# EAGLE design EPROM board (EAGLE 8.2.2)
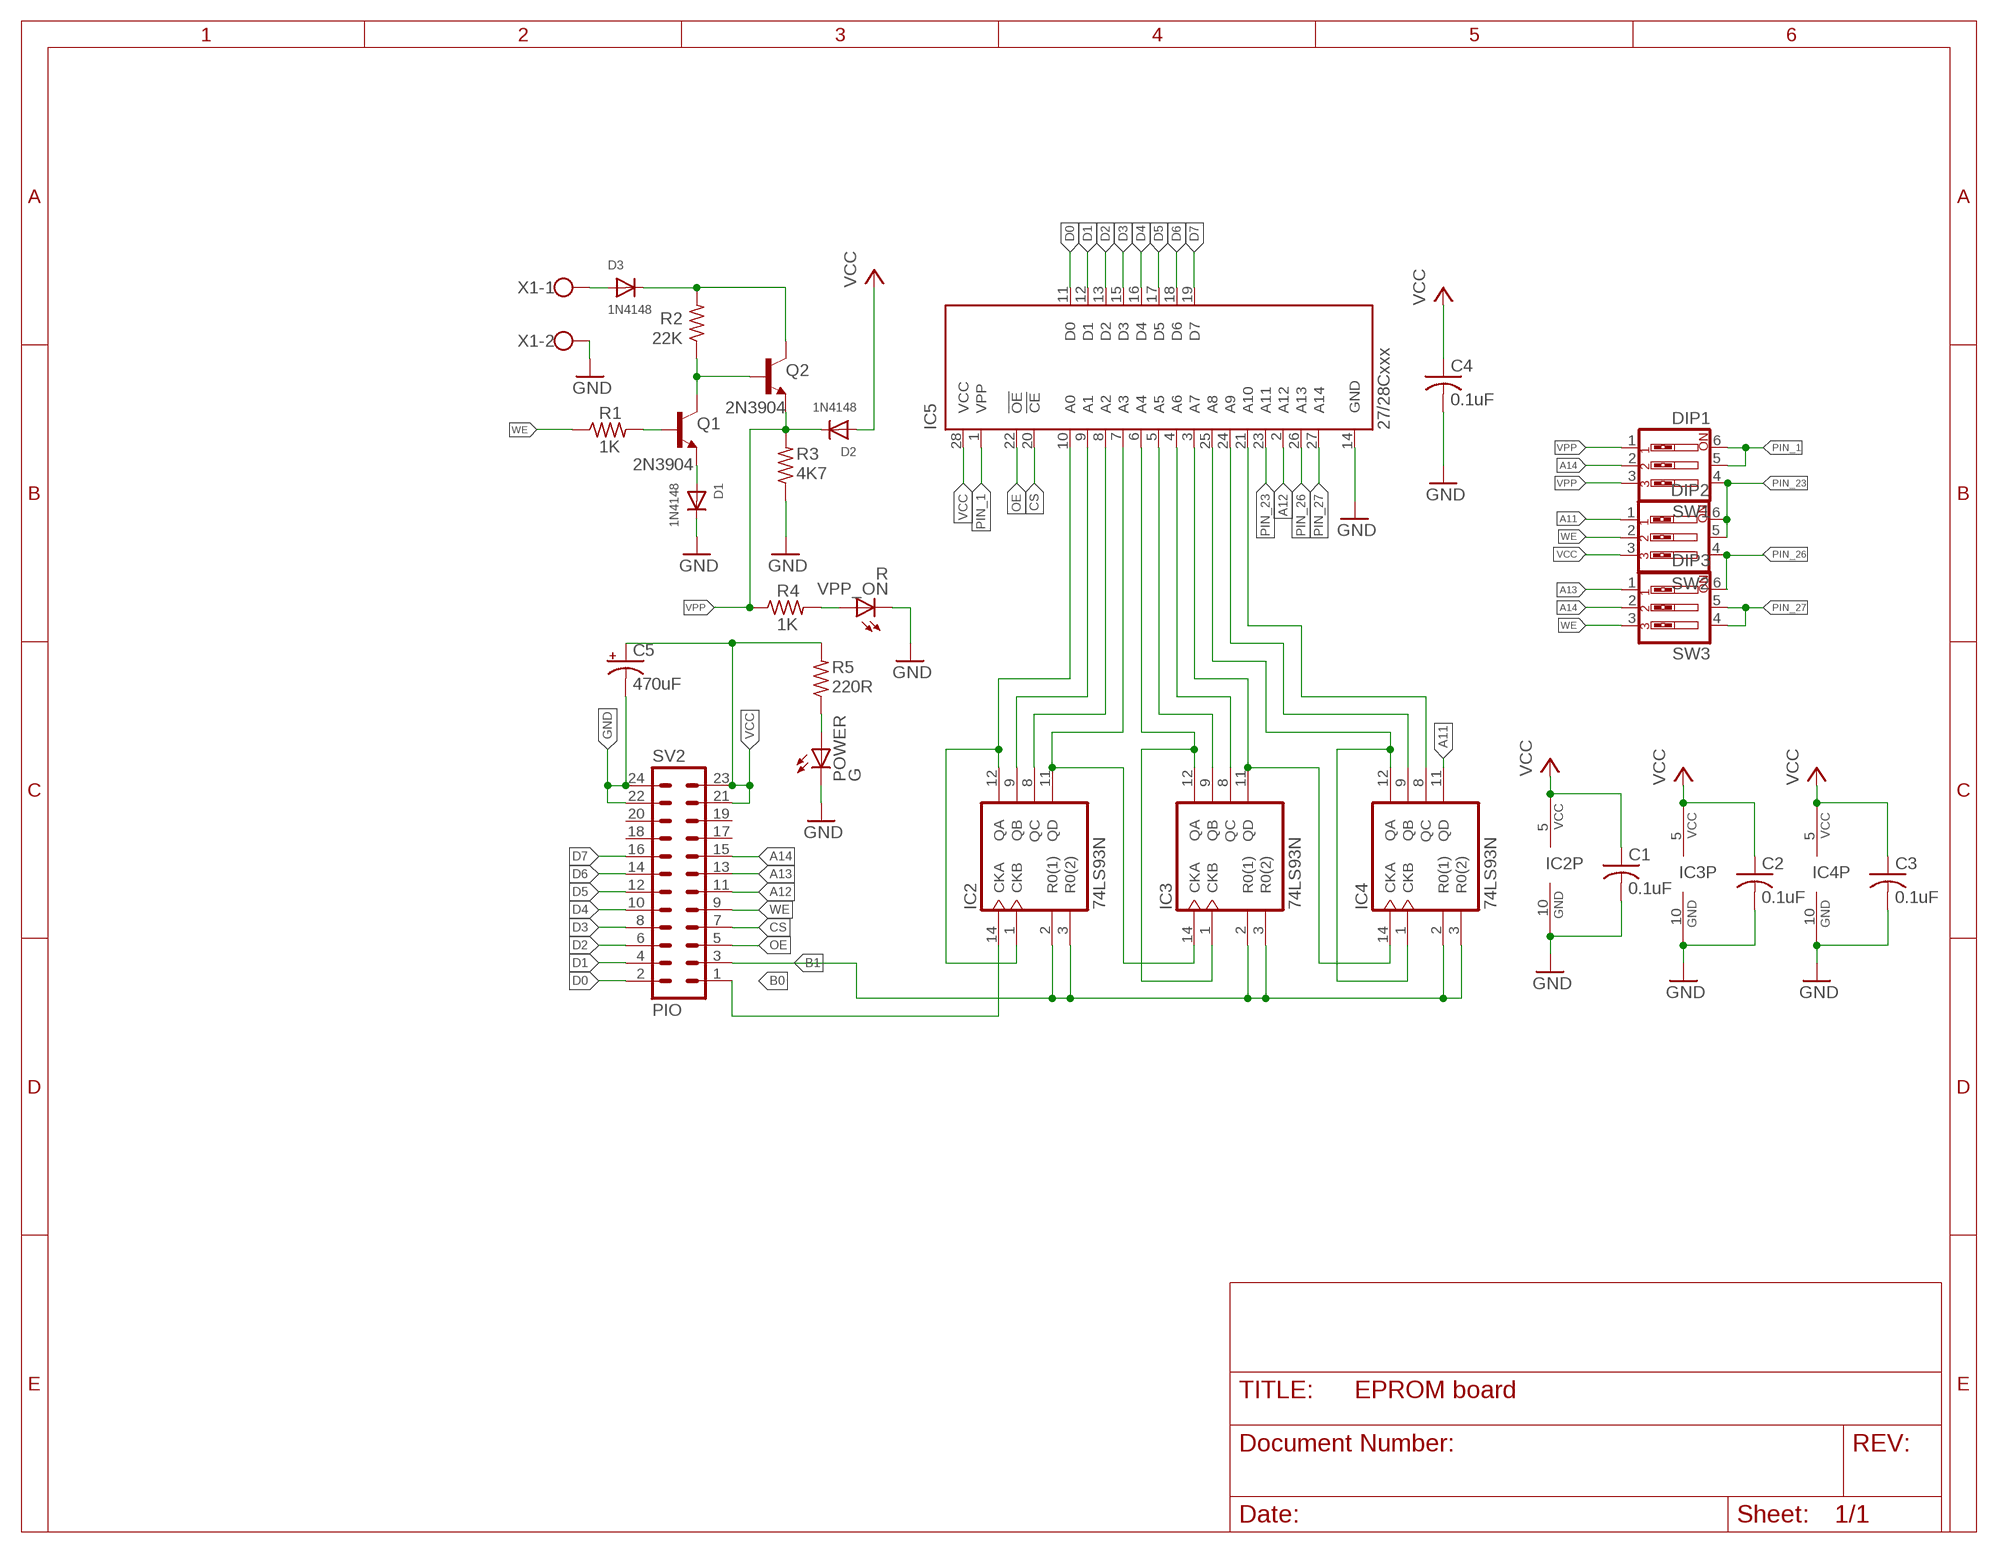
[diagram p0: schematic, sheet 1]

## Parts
C1  0.1uF  C-US025-025X050  [C025-025X050]
C2  0.1uF  C-US025-025X050  [C025-025X050]
C3  0.1uF  C-US025-025X050  [C025-025X050]
C4  0.1uF  C-US025-025X050  [C025-025X050]
C5  470uF  CPOL-USE5-6  [E5-6]
D1  1N4148  DIODEDO-1N4148  [DO-1N4148]
D2  1N4148  DIODEDO-1N4148  [DO-1N4148]
D3  1N4148  DIODEDO-1N4148  [DO-1N4148]
IC2  74LS93N  [DIL14]
IC3  74LS93N  [DIL14]
IC4  74LS93N  [DIL14]
IC5  27/28Cxxx  27C256P  [DIL28-6]
POWER  G  LED5MM  [LED5MM]
Q1  2N3904  [TO92]
Q2  2N3904  [TO92]
R1  1K  R-US_0204/7  [0204/7]
R2  22K  R-US_0204/7  [0204/7]
R3  4K7  R-US_0204/7  [0204/7]
R4  1K  R-US_0204/7  [0204/7]
R5  220R  R-US_0204/7  [0204/7]
SV2  PIO  MA12-2W  [MA12-2W]
SW1  DIP1  SW_DIP-3  [EDG-03]
SW2  DIP2  SW_DIP-3  [EDG-03]
SW3  DIP3  SW_DIP-3  [EDG-03]
VPP_ON  R  LED5MM  [LED5MM]
X1  W237-102  [W237-102]

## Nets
A11: IC4.11(QD) SW2.1
A12: IC5.2(A12) SV2.11
A13: SV2.13 SW3.1
A14: SV2.15 SW1.2 SW3.2
B0: IC2.14(CKA) SV2.1
B1: IC2.2(R0(1)) IC2.3(R0(2)) IC3.2(R0(1)) IC3.3(R0(2)) IC4.2(R0(1)) IC4.3(R0(2)) SV2.3
CS: IC5.20(!CE) SV2.7
D0: IC5.11(D0) SV2.2
D1: IC5.12(D1) SV2.4
D2: IC5.13(D2) SV2.6
D3: IC5.15(D3) SV2.8
D4: IC5.16(D4) SV2.10
D5: IC5.17(D5) SV2.12
D6: IC5.18(D6) SV2.14
D7: IC5.19(D7) SV2.16
GND: C1.2 C2.2 C3.2 C4.2 C5.- D1.C IC2.10(GND) IC3.10(GND) IC4.10(GND) IC5.14(GND) POWER.K(C) R3.1 SV2.22 SV2.24 VPP_ON.K(C) X1.2
N$1: IC2.1(CKB) IC2.12(QA) IC5.10(A0)
N$2: IC2.9(QB) IC5.9(A1)
N$3: IC2.8(QC) IC5.8(A2)
N$4: IC2.11(QD) IC3.14(CKA) IC5.7(A3)
N$5: IC3.1(CKB) IC3.12(QA) IC5.6(A4)
N$6: IC3.9(QB) IC5.5(A5)
N$7: IC3.8(QC) IC5.4(A6)
N$8: IC3.11(QD) IC4.14(CKA) IC5.3(A7)
N$9: IC4.1(CKB) IC4.12(QA) IC5.25(A8)
N$10: IC4.9(QB) IC5.24(A9)
N$11: IC4.8(QC) IC5.21(A10)
N$12: POWER.A R5.1
N$13: Q1.2(B) R1.2
N$14: D1.A Q1.3(E)
N$15: Q1.1(C) Q2.2(B) R2.1
N$16: D3.A X1.1
N$17: D3.C Q2.1(C) R2.2
N$18: R4.2 VPP_ON.A
OE: IC5.22(!OE) SV2.5
PIN_1: IC5.1(VPP) SW1.5 SW1.6
PIN_23: IC5.23(A11) SW1.4 SW2.5 SW2.6
PIN_26: IC5.26(A13) SW2.4 SW3.6
PIN_27: IC5.27(A14) SW3.4 SW3.5
VCC: C1.1 C2.1 C3.1 C4.1 C5.+ D2.A IC2.5(VCC) IC3.5(VCC) IC4.5(VCC) IC5.28(VCC) R5.2 SV2.21 SV2.23 SW2.3
VPP: D2.C Q2.3(E) R3.2 R4.1 SW1.1 SW1.3
WE: R1.1 SV2.9 SW2.2 SW3.3
Unconnected: SV2.17 SV2.18 SV2.19 SV2.20

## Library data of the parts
C1-C4 = rcl:C-US: CAPACITOR, American symbol
C5 = rcl:CPOL-US: POLARIZED CAPACITOR, American symbol
D1-D3 = adafruit:DIODE: Diode
IC2-IC4 = 74xx-us:74*93: Decade, divide by twelve and binary COUNTER
IC5 = microchip:27*256: CMOS EPROM 256 K (32 K x 8), low voltage; MF: Arrow Electronics; MPN: M27C256B15F1; OC_FARNELL: 1125431; OC_NEWARK: 93K7335
POWER VPP_ON = led:LED: LED
Q1 Q2 = transistor-npn:2N3904: NPN Transistor
R1-R5 = rcl:R-US_: RESISTOR, American symbol
SV2 = con-lstb:MA12-2W: PIN HEADER; OC_FARNELL: unknown; OC_NEWARK: unknown
SW1-SW3 = special:SW_DIP-3: DIP SWITCH
X1 = con-wago-500:W237-102: WAGO SCREW CLAMP; MPN: 237-102; OC_FARNELL: unknown; OC_NEWARK: 70K9898

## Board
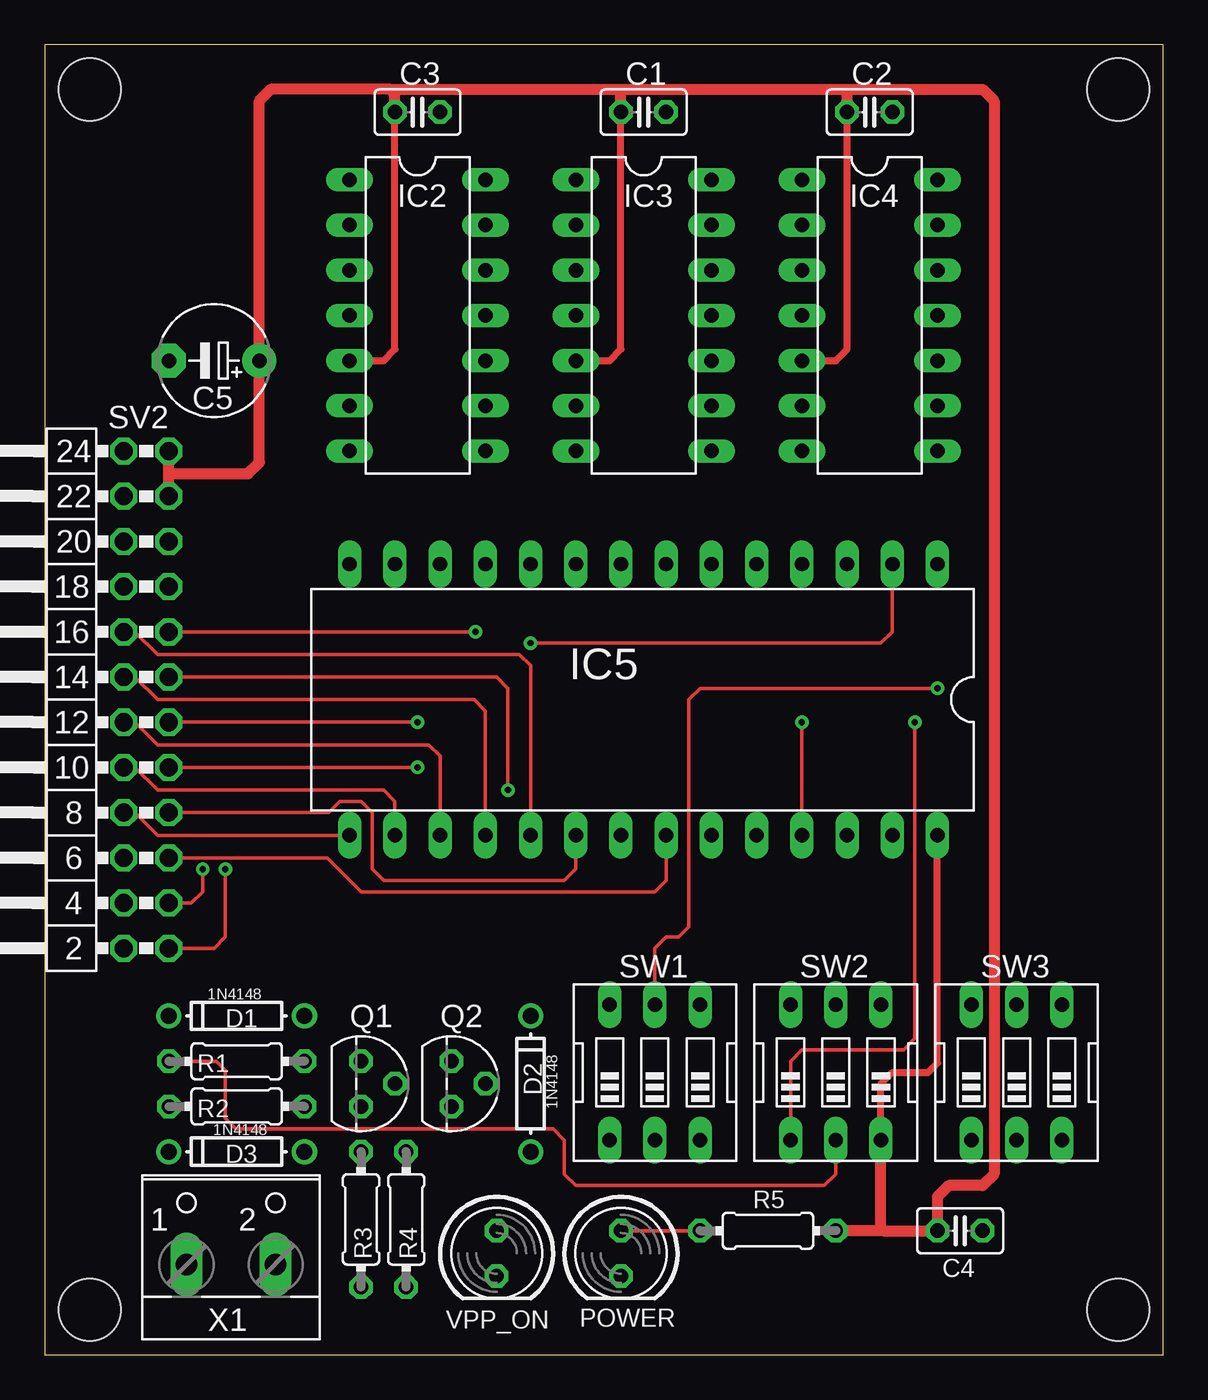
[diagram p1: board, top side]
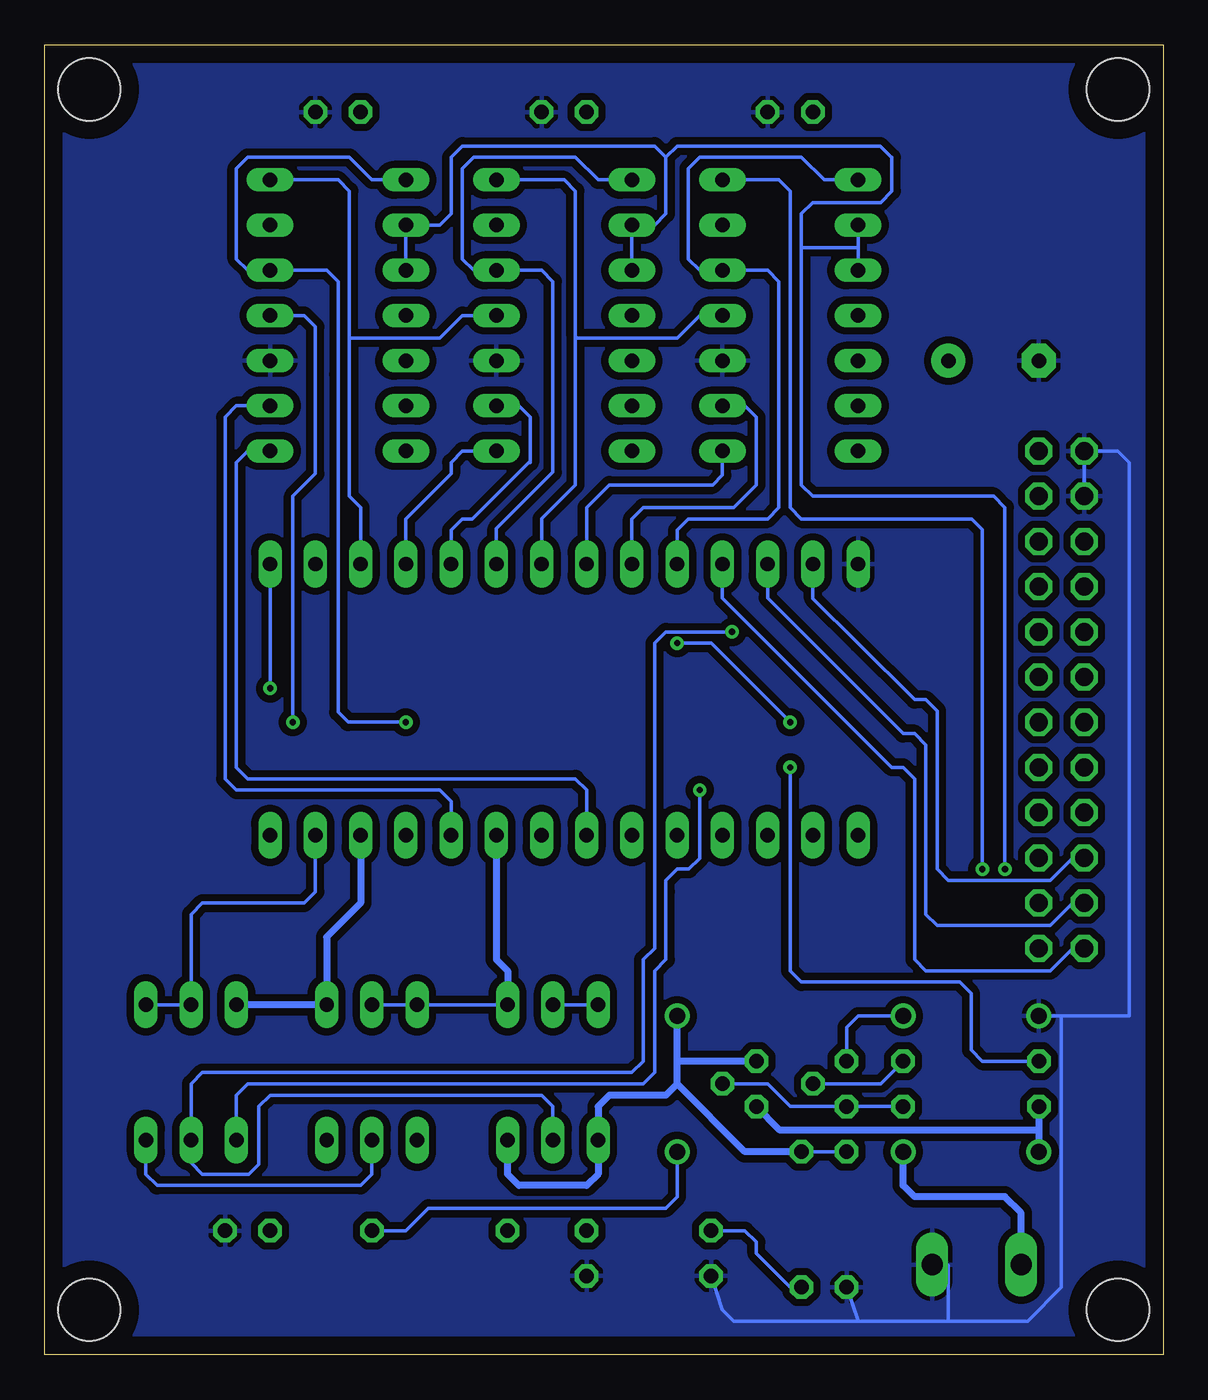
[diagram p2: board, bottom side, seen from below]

Size 62.84 x 73.65 mm. Coordinates in mm from the lower left corner, seen from the top.
Outline: 0,0 62.84,0 62.84,73.65 0,73.65 0,0
Copper layers (1*16): Top 0.035mm / dielectric 1.5mm / Bottom 0.035mm
Design rules "default": minimum track width 6mil, minimum drill 0.35mm, track to track 6mil, track to pad 6mil, pad to pad 6mil, via to via 6mil, smd to smd 6mil, copper to edge 40mil, drill to drill 6mil, minimum pad ring 10mil, minimum via ring 8mil, stop-mask expansion 4mil, vias tented up to drill 0mil, thermal gap 10mil
Holes 3.5 mm at 2.54,2.54 2.54,71.12 60.33,2.54 60.33,71.12

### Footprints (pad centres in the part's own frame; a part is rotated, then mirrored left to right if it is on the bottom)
C025-025X050 = drill 0.813 octagon: 1 -1.27,0; 2 1.27,0
E5-6 = drill 0.813 pad 1.905: + -2.54,0 | drill 0.813 pad 1.905 octagon: - 2.54,0
DO-1N4148 = drill 0.9: A -3.81,0; C 3.81,0
DIL14 = drill 0.813 long: 1 -7.62,-3.81; 2 -5.08,-3.81; 3 -2.54,-3.81; 4 0,-3.81; 5 2.54,-3.81; 6 5.08,-3.81; 7 7.62,-3.81; 8 7.62,3.81; 9 5.08,3.81; 10 2.54,3.81; 11 0,3.81; 12 -2.54,3.81; 13 -5.08,3.81; 14 -7.62,3.81
DIL28-6 = drill 0.813 long: 1 -16.51,-7.62; 2 -13.97,-7.62; 3 -11.43,-7.62; 4 -8.89,-7.62; 5 -6.35,-7.62; 6 -3.81,-7.62; 7 -1.27,-7.62; 8 1.27,-7.62; 9 3.81,-7.62; 10 6.35,-7.62; 11 8.89,-7.62; 12 11.43,-7.62; 13 13.97,-7.62; 14 16.51,-7.62; 15 16.51,7.62; 16 13.97,7.62; 17 11.43,7.62; 18 8.89,7.62; 19 6.35,7.62; 20 3.81,7.62; 21 1.27,7.62; 22 -1.27,7.62; 23 -3.81,7.62; 24 -6.35,7.62; 25 -8.89,7.62; 26 -11.43,7.62; 27 -13.97,7.62; 28 -16.51,7.62
LED5MM = drill 0.813 octagon: A -1.27,0; K 1.27,0
TO92 = drill 0.813 octagon: 1 1.27,0; 2 0,1.905; 3 -1.27,0
0204/7 = drill 0.813 octagon: 1 -3.81,0; 2 3.81,0
MA12-2W = drill 1.016 octagon: 1 -13.97,-1.27; 2 -13.97,1.27; 3 -11.43,-1.27; 4 -11.43,1.27; 5 -8.89,-1.27; 6 -8.89,1.27; 7 -6.35,-1.27; 8 -6.35,1.27; 9 -3.81,-1.27; 10 -3.81,1.27; 11 -1.27,-1.27; 12 -1.27,1.27; 13 1.27,-1.27; 14 1.27,1.27; 15 3.81,-1.27; 16 3.81,1.27; 17 6.35,-1.27; 18 6.35,1.27; 19 8.89,-1.27; 20 8.89,1.27; 21 11.43,-1.27; 22 11.43,1.27; 23 13.97,-1.27; 24 13.97,1.27
EDG-03 = drill 0.813 long: 1 -2.54,-3.81; 2 0,-3.81; 3 2.54,-3.81; 4 2.54,3.81; 5 0,3.81; 6 -2.54,3.81
W237-102 = drill 1.194 long: 1 -2.5,-1.27; 2 2.5,-1.27

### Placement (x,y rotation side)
C1  33.66,69.85 0 top
C2  46.35,69.85 0 top
C3  20.95,69.85 0 top
C4  51.44,6.99 0 top
C5  9.53,55.88 180 top
D1  10.79,19.05 180 top
D2  27.3,15.24 90 top
D3  10.79,11.43 180 top
IC2  20.95,58.42 270 top
IC3  33.66,58.42 270 top
IC4  46.35,58.42 270 top
IC5  33.66,36.83 180 top
POWER  32.38,5.71 270 top
Q1  17.78,15.24 270 top
Q2  22.86,15.24 270 top
R1  10.79,16.51 0 top
R2  10.79,13.97 180 top
R3  17.78,7.62 90 top
R4  20.32,7.62 270 top
R5  40.64,6.99 0 top
SV2  5.71,36.83 90 top
SW1  34.29,15.88 0 top
SW2  44.45,15.88 0 top
SW3  54.61,15.88 0 top
VPP_ON  25.4,5.71 270 top
X1  10.48,6.35 0 top

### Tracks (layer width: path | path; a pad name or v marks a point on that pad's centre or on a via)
A11  (via drill 0.35)
  Top 0.2: SW2.1 41.91,16.51 42.55,17.14 48.26,17.14 48.9,17.78 v48.9,35.56
  Bottom 0.2: v48.9,35.56 48.9,48.26 47.62,49.53 47.62,57.78 48.26,58.42 IC4.11
A12  (via drill 0.35)
  Top 0.2: SV2.11 v20.95,35.56 | IC5.2 47.62,40.64 46.99,40.01 29.07,40.01
  Top 0.203: 29.07,40.01 v27.3,40.01
  Bottom 0.203: v27.3,40.01 25.4,40.01 v20.95,35.56
A13  (via drill 0.35)
  Top 0.2: v26.04,31.75 26.04,37.47 25.4,38.1 SV2.13
  Bottom 0.2: SW3.1 52.07,14.61 51.44,15.24 29.21,15.24 28.57,15.88 28.57,21.59 27.94,22.23 27.94,26.04 | 27.3,27.3 26.67,27.3 | 26.04,27.92 v26.04,31.75
  Bottom 0.203: 27.94,26.04 27.94,26.67 27.3,27.3 | 26.67,27.3 26.65,27.3 26.04,27.92
A14  (via drill 0.35)
  Top 0.2: v24.22,40.64 SV2.15
  Bottom 0.2: SW1.2 34.29,13.97 34.92,14.61 50.16,14.61 50.8,13.97 50.8,10.72 51.36,10.16 53.98,10.16 54.61,10.79 SW3.2 54.61,15.24 53.98,15.88 29.84,15.88 29.21,16.51 29.21,22.23 28.57,22.86 28.57,40.01 27.94,40.64 v24.22,40.64 24.13,40.64
B0  (via drill 0.35)
  Top 0.2: SV2.1 9.53,22.86 10.16,23.5 v10.16,27.3
  Bottom 0.2: IC2.14 21.59,66.04 20.95,65.41 20.95,47.62 20.32,46.99 10.75,46.99 10.16,46.4 v10.16,27.3
B1  (via drill 0.35)
  Top 0.2: SV2.3 8.26,25.4 8.89,26.04 v8.89,27.3
  Bottom 0.2: v8.89,27.3 8.89,47.62 9.53,48.26 19.68,48.26 20.32,48.9 20.32,62.23 | 27.94,67.31 28.57,67.94 39.37,67.94 40.01,67.31 40.01,64.14 40.64,63.5 IC4.2 IC4.3 | 27.94,67.31 27.94,64.14 28.57,63.5 IC3.2 IC3.3 | 27.94,67.31 27.3,67.94 15.9,67.94 15.26,67.31 15.24,67.31 15.24,65.41 15.88,64.77 19.68,64.77 20.32,64.14 20.32,62.23 | IC2.3 17.14,62.23 | 17.14,62.23 IC2.2 | 17.14,62.23 20.32,62.23
CS
  Top 0.2: IC5.20 29.84,27.3 29.21,26.67 19.05,26.67 18.41,27.3 18.41,30.48 17.78,31.11 16.59,31.11 15.95,30.48 SV2.7
D0
  Bottom 0.2: IC5.11 24.77,42.55 15.24,33.02 14.61,33.02 13.97,32.38 13.97,22.23 13.34,21.59 6.35,21.59 5.08,22.86 SV2.2
D1
  Bottom 0.2: IC5.12 22.23,42.55 14.61,34.92 13.97,34.92 13.34,34.29 13.34,24.77 12.7,24.13 6.35,24.13 5.08,25.4 SV2.4
D2
  Bottom 0.2: IC5.13 19.68,42.52 17.14,39.98 17.12,39.98 13.97,36.83 13.34,36.83 12.7,36.2 12.7,27.3 12.06,26.67 6.35,26.67 5.08,27.94 SV2.6
D3
  Top 0.2: IC5.15 6.35,29.21 5.08,30.48 SV2.8
D4
  Top 0.2: IC5.16 19.68,31.11 19.05,31.75 6.35,31.75 5.08,33.02 SV2.10
D5
  Top 0.2: IC5.17 22.23,33.66 21.59,34.29 6.35,34.29 5.08,35.56 SV2.12
D6
  Top 0.2: IC5.18 24.77,36.2 24.13,36.83 6.35,36.83 5.08,38.1 SV2.14
D7
  Top 0.2: IC5.19 27.3,38.73 26.67,39.37 6.35,39.37 5.08,40.64 SV2.16
GND
  Bottom 0.2: 4.45,50.75 SV2.22 | 4.45,50.75 SV2.24 | VPP_ON.K 24.77,2.54 24.13,1.91 17.11,1.91 | 17.11,1.91 12.06,1.91 | 12.06,1.91 12.06,5.04 X1.2 | R3.1 17.14,1.94 17.11,1.91 | 12.06,1.91 7.62,1.91 5.71,3.81 5.71,19.02 5.69,19.05 | 5.69,19.05 D1.C | 5.69,19.05 1.91,19.05 1.91,50.16 2.54,50.8 4.39,50.8 4.45,50.75
  pour Bottom (isolate 0.406): 0,0 0,73.66 62.87,73.66 62.87,0
N$1
  Bottom 0.2: IC2.1 19.05,66.04 20.32,67.31 26.04,67.31 26.67,66.67 26.67,61.59 26.04,60.96 IC2.12 22.23,60.96 21.59,60.33 21.59,47.62 22.23,46.99 26.67,46.99 27.3,46.35 IC5.10
N$2
  Bottom 0.2: IC5.9 29.84,46.99 29.21,47.62 24.13,47.62 22.86,48.9 22.86,52.7 23.5,53.34 IC2.9
N$3
  Bottom 0.2: IC5.8 32.38,47.62 31.11,48.9 25.32,48.9 24.77,49.45 IC2.8
N$4
  Bottom 0.2: IC2.11 26.04,58.42 27.3,57.15 32.91,57.15 33.02,57.26 | 34.29,66.04 IC3.14 33.66,66.04 33.02,65.41 33.02,57.26 | 33.02,57.26 33.02,48.9 33.03,48.9 34.92,47 IC5.7
N$5
  Bottom 0.2: IC3.1 31.75,66.04 33.02,67.31 38.73,67.31 39.37,66.67 39.37,61.59 38.73,60.96 IC3.12 34.92,60.96 34.29,60.33 34.29,49.62 37.47,46.44 IC5.6
N$6
  Bottom 0.2: IC5.5 40.01,46.35 39.37,46.99 38.82,46.99 35.65,50.16 35.56,50.16 35.56,52.7 36.2,53.34 IC3.9
N$7
  Bottom 0.2: IC5.4 42.55,46.99 40.01,49.53 40.01,50.16 39.37,50.8 IC3.8
N$8
  Bottom 0.2: IC5.3 45.09,47.62 45.72,48.26 45.72,57.22 | IC3.11 39.37,58.42 40.64,57.15 45.65,57.15 45.72,57.22 | 45.72,57.22 45.72,65.41 46.35,66.04 IC4.14
N$9  (via drill 0.35)
  Top 0.2: v42.55,35.56 IC5.25
  Bottom 0.2: IC4.1 44.45,66.04 45.72,67.31 51.44,67.31 52.07,66.67 52.07,61.59 51.44,60.96 IC4.12 46.99,60.96 | 46.35,55.1 46.35,36.12 45.79,35.56 v42.55,35.56
  Bottom 0.203: 46.99,60.96 46.35,60.33 46.35,55.1
N$10
  Bottom 0.2: IC4.9 52.07,53.34 52.7,52.7 52.7,32.38 52.07,31.75 40.64,31.75 40.01,31.11 IC5.24
N$11
  Bottom 0.2: IC5.21 32.38,31.75 33.02,32.38 51.44,32.38 52.07,33.02 52.07,50.16 51.44,50.8 IC4.8
N$12
  Top 0.2: POWER.A R5.1
N$13
  Bottom 0.2: R1.2 15.88,15.24 Q1.2
N$14
  Bottom 0.2: Q1.3 17.78,18.41 17.14,19.05 D1.A
N$15
  Bottom 0.2: R2.1 Q1.1 20.95,13.97 22.23,15.24 Q2.2
N$16
  Bottom 0.406: X1.1 7.98,7.98 8.89,8.89 13.97,8.89 14.61,9.53 D3.A
N$17
  Bottom 0.406: 6.99,12.64 D3.C | 6.99,12.64 7.05,12.7 | 6.99,12.64 21.53,12.64 Q2.1 | R2.2 6.99,12.64
N$18
  Bottom 0.2: R4.2 20.95,3.81 22.86,5.71 22.86,6.35 23.5,6.99 VPP_ON.A
OE
  Top 0.2: IC5.22 34.92,26.67 34.29,26.04 17.79,26.04 15.88,27.94 SV2.5
PIN_1  (via drill 0.35)
  Top 0.2: SW1.5 34.29,21.59 | v50.16,37.47 36.83,37.47 36.2,36.83 36.2,24.05
  Top 0.203: 34.29,21.59 34.29,22.86 34.92,23.5 35.63,23.5 36.2,24.05
  Bottom 0.2: SW1.6 SW1.5 | IC5.1 v50.16,37.47
PIN_23
  Bottom 0.2: SW1.4 SW2.6 SW2.5
  Bottom 0.406: IC5.23 37.47,22.23 36.83,21.59 SW1.4
PIN_26
  Bottom 0.406: IC5.26 45.09,25.4 46.99,23.5 SW2.4 SW3.6
PIN_27
  Bottom 0.2: SW3.4 SW3.5 54.61,24.77
  Bottom 0.203: 54.61,24.77 53.98,25.4 48.26,25.4 47.62,26.04 IC5.27
VCC
  Top 0.2: 19.68,69.7 C3.1
  Top 0.406: IC2.5 19.05,55.88 19.68,56.52 19.68,69.7 | IC3.5 31.75,55.88 32.38,56.52 C1.1 | IC4.5 44.45,55.88 45.09,56.52 C2.1 | IC5.28 50.16,16.39 49.65,15.88 47.62,15.88 46.99,15.24 SW2.3
  Top 0.61: 19.53,69.85 19.68,69.7 | 47.08,6.99 C4.1 50.16,8.89 50.8,9.53 52.7,9.53 53.34,10.16 53.34,70.48 52.7,71.12 45.09,71.12 | 47.08,6.99 R5.2 | SW2.3 46.99,7.08 47.08,6.99 | SV2.21 6.99,49.53 | 6.99,49.53 SV2.23 | 6.99,49.53 11.43,49.53 12.06,50.16 C5.+ 12.06,70.48 12.7,71.12 19.43,71.12 | 32.38,71.12 45.09,71.12 | 19.43,71.12 32.38,71.12 | C2.1 45.09,71.11 45.09,71.12 | C1.1 32.38,71.12 | C3.1 19.68,70.86 19.43,71.12
  Bottom 0.2: R5.2 42.55,6.99 41.27,8.26 27.94,8.26 27.3,8.89 D2.A
VPP
  Bottom 0.2: R3.2 R4.1
  Bottom 0.406: R4.1 23.5,11.43 27.3,15.24 | 27.3,15.24 27.3,16.48 | 27.3,16.48 D2.C | Q2.3 27.27,16.51 27.3,16.48 | 27.3,15.24 27.94,14.61 31.11,14.61 31.75,13.97 SW1.1 31.75,10.16 32.38,9.53 36.2,9.53 36.83,10.16 SW1.3
WE  (via drill 0.35)
  Top 0.2: R1.1 9.66,16.51 10.16,16.01 10.16,13.29 10.76,12.7 28.58,12.7 29.21,12.07 29.21,10.16 29.84,9.53 43.81,9.53 44.45,10.16 SW2.2 | SV2.9 v20.95,33.02
  Bottom 0.2: SW2.2 44.45,10.16 45.09,9.53 56.52,9.53 57.15,10.16 SW3.3 | R1.1 7.01,16.53 7.03,16.51 10.16,16.51 10.79,17.14 10.79,20.32 11.43,20.95 20.32,20.95 20.95,21.59 v20.95,33.02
